(* Logix 5000 AddOnInstructionDefinition export OM_AZ_MONITOR; software revision 30.00 *)

ADD_ON_INSTRUCTION OM_AZ_MONITOR   (* revision 1.3, vendor ORIENTALMOTOR CO.,LTD. *)
// Revision note:
// Implicit message based on AZD-AEP,-CEP and -KEP.
// Help:
// This AOI is used to monitor the present alarm, feedback position, feedback speed, command position, torque monitor, CST operating current, information, driver temperature, motor temperature, cumulative load and tripmeter.
// The driver temperature, motor temperature, cumulative load monitor, and tripmeter are used as assignable monitor setting parameters as an initial value. Assignable monitor settings can also be changed to check for other parameters.
VAR_IN_OUT
   ImplicitMSGinput : INT[28]; {required}   // Implicit message Input (driver->scanner)
        [0]   // Remote I/O (R-OUT)
        [0].0   // R-OUT0
        [0].1   // R-OUT1
        [0].2   // R-OUT2
        [0].3   // R-OUT3
        [0].4   // R-OUT4
        [0].5   // R-OUT5
        [0].6   // R-OUT6
        [0].7   // R-OUT7
        [0].8   // R-OUT8
        [0].9   // R-OUT9
        [0].10   // R-OUT10
        [0].11   // R-OUT11
        [0].12   // R-OUT12
        [0].13   // R-OUT13
        [0].14   // R-OUT14
        [0].15   // R-OUT15
        [1]   // Operation data number selection_R
        [1].0   // M0_R
        [1].1   // M1_R
        [1].2   // M2_R
        [1].3   // M3_R
        [1].4   // M4_R
        [1].5   // M5_R
        [1].6   // M6_R
        [1].7   // M7_R
        [1].8   // Reserved
        [1].9   // Reserved
        [1].10   // Reserved
        [1].11   // Reserved
        [1].12   // Reserved
        [1].13   // Reserved
        [1].14   // Reserved
        [1].15   // Reserved
        [2]   // Fixed I/O (OUT)
        [2].0   // SEQ-BSY
        [2].1   // MOVE
        [2].2   // IN-POS
        [2].3   // START_R
        [2].4   // HOME-END
        [2].5   // READY
        [2].6   // DCMD-RDY
        [2].7   // ALM-A
        [2].8   // TRIG_R
        [2].9   // TRIG-MODE_R
        [2].10   // SET-ERR
        [2].11   // EXE-ERR
        [2].12   // DCMD-FULL
        [2].13   // STOP_R
        [2].14   // ETO-MON
        [2].15   // TLC
        [3]   // Present alarm
        [4]   // Feedback position (lower)
        [5]   // Feedback position (upper)
        [6]   // Feedback speed [Hz] (lower)
        [7]   // Feedback speed [Hz] (upper)
        [8]   // Command position (lower)
        [9]   // Command position (upper)
        [10]   // Torque monitor
        [11]   // CST operating current
        [12]   // Information (lower)
        [13]   // Information (upper)
        [14]   // Reserved
        [15]   // Read parameter ID_R
        [16]   // Read/write status
        [16].0   // Reserved
        [16].1   // Reserved
        [16].2   // Reserved
        [16].3   // Reserved
        [16].4   // Reserved
        [16].5   // Reserved
        [16].6   // Reserved
        [16].7   // RD-ERR
        [16].8   // WR-END
        [16].9   // SYS-BSY
        [16].10   // Reserved
        [16].11   // WR-SET-ERR
        [16].12   // WR-IF-ERR
        [16].13   // WR-NV-ERR
        [16].14   // WR-EXE-ERR
        [16].15   // WR-ERR
        [17]   // Write parameter ID_R
        [18]   // Read data (lower)
        [19]   // Read data (upper)
        [20]   // Assignable monitor 0 (lower)
        [21]   // Assignable monitor 0 (upper)
        [22]   // Assignable monitor 1 (lower)
        [23]   // Assignable monitor 1 (upper)
        [24]   // Assignable monitor 2 (lower)
        [25]   // Assignable monitor 2 (upper)
        [26]   // Assignable monitor 3 (lower)
        [27]   // Assignable monitor 3 (upper)
END_VAR
VAR_OUTPUT
   Read_Present_alarm : INT; {visible}   // Alarm code monitor[Hex]
   Read_Feedback_position : DINT; {visible}   // Feedback position monitor[step]
   Read_Feedback_speed : DINT; {visible}   // Feedback speed monitor[Hz]
   Read_Command_position : DINT; {visible}   // Command position monitor[step]
   Read_Torque_monitor : INT; {visible}   // Torque monitor as a percentage of the maximum holding torque[1=0.1%]
   Read_CST_operating_current : INT; {visible}   // Operation current monitor in alpha control mode(CST) (1=0.1%)
   Read_Information : DINT; {visible}   // Information monitor before an alarm is generated.
   Read_Driver_temperature : DINT; {visible}   // Driver temperature monitor(1=0.1deg)
   Read_Motor_temperature : DINT; {visible}   // Motor temperature monitor(1=0.1deg)
   Read_Cumulative_load_monitor : DINT; {visible}   // Cumulative load monitor
   Read_Tripmeter : DINT; {visible}   // Travel distance monitor[x1000rev]
END_VAR
VAR
   temp : INT[25]; {access None}
END_VAR

ROUTINE Logic   (* ladder *)
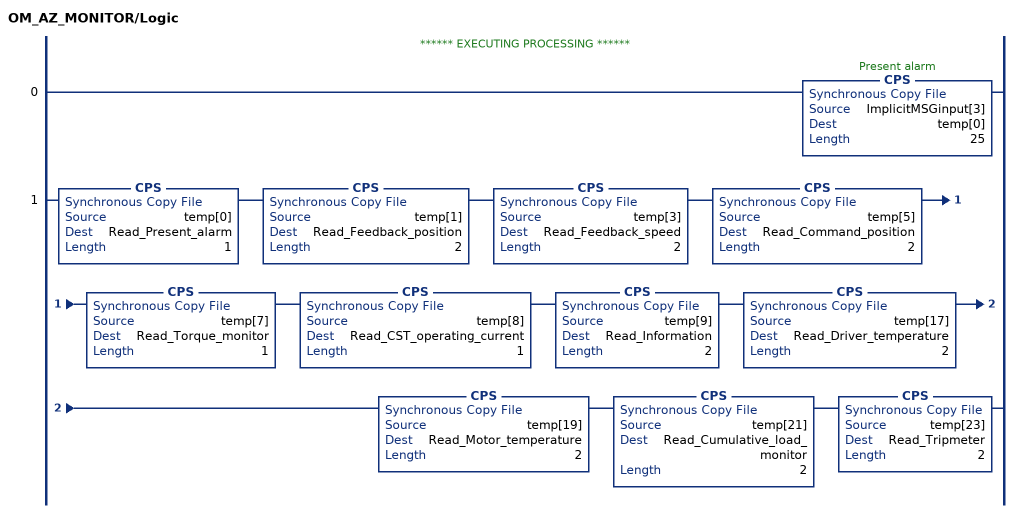
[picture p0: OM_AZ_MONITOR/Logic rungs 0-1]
   // ****** EXECUTING PROCESSING ******
   0: CPS(ImplicitMSGinput[3],temp[0],25);
   1: CPS(temp[0],Read_Present_alarm,1)CPS(temp[1],Read_Feedback_position,2)CPS(temp[3],Read_Feedback_speed,2)CPS(temp[5],Read_Command_position,2)CPS(temp[7],Read_Torque_monitor,1)CPS(temp[8],Read_CST_operating_current,1)CPS(temp[9],Read_Information,2)CPS(temp[17],Read_Driver_temperature,2)CPS(temp[19],Read_Motor_temperature,2)CPS(temp[21],Read_Cumulative_load_monitor,2)CPS(temp[23],Read_Tripmeter,2);
END_ROUTINE
END_ADD_ON_INSTRUCTION
